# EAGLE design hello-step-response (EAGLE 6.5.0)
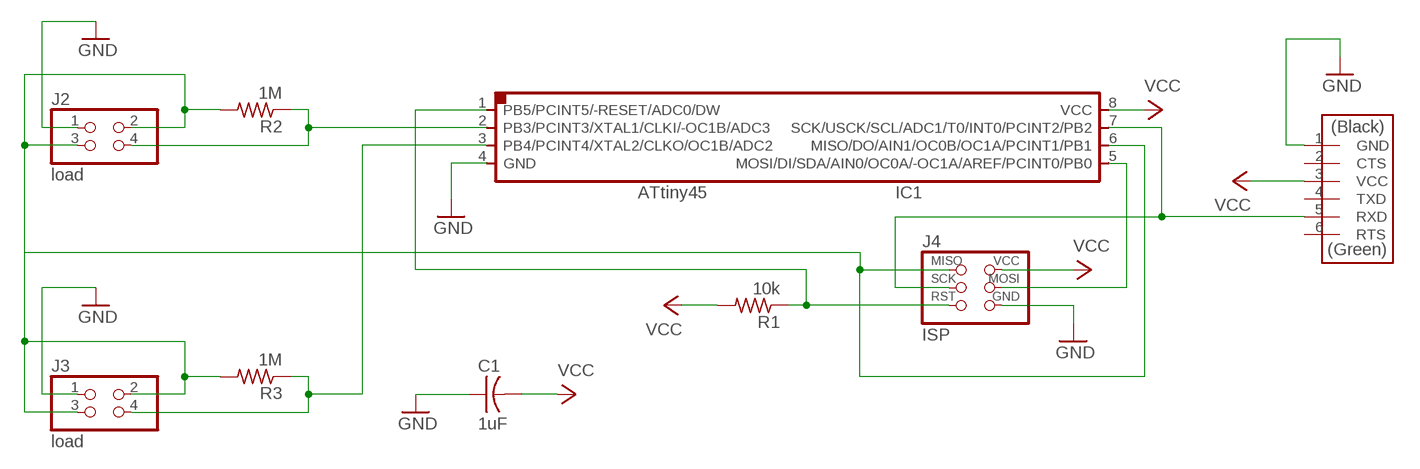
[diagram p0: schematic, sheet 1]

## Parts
C1  1uF  CAP-US1206FAB  [C1206FAB]
IC1  ATTINY45  ATTINY45SI  [SOIC8]
J1  FTDI  FTDI-SMD-HEADER  [1X06SMD]
J2  load  PINHD-2X2-SMD  [2X02SMD]
J3  load  PINHD-2X2-SMD  [2X02SMD]
J4  ISP  AVRISPSMD  [2X03SMD]
R1  10k  RES-US1206FAB  [R1206FAB]
R2  1M  RES-US1206FAB  [R1206FAB]
R3  1M  RES-US1206FAB  [R1206FAB]

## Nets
GND: C1.1 IC1.4(GND) J1.1(GND) J2.1 J3.1 J4.6(GND)
MISO: IC1.6(MISO/DO/AIN1/OC0B/OC1A/PCINT1/PB1) J2.2 J2.3 J3.2 J3.3 J4.1(MISO) R2.2 R3.2
MOSI: IC1.5(MOSI/DI/SDA/AIN0/OC0A/-OC1A/AREF/PCINT0/PB0) J4.4(MOSI)
N$5: IC1.2(PB3/PCINT3/XTAL1/CLKI/-OC1B/ADC3) J2.4 R2.1
N$6: IC1.3(PB4/PCINT4/XTAL2/CLKO/OC1B/ADC2) J3.4 R3.1
RST: IC1.1(PB5/PCINT5/-RESET/ADC0/DW) J4.5(RST) R1.1
SCK: IC1.7(SCK/USCK/SCL/ADC1/T0/INT0/PCINT2/PB2) J1.5(RXD) J4.3(SCK)
VCC: C1.2 IC1.8(VCC) J1.3(VCC) J4.2(VCC) R1.2
Unconnected: J1.2(CTS) J1.4(TXD) J1.6(RTS)

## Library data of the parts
C1 = fab:CAP-US
IC1 = fab:ATTINY45
J1 = fab:FTDI-SMD-HEADER
J2 J3 = fab:PINHD-2X2-SMD
J4 = fab:AVRISP
R1-R3 = fab:RES-US: Resistor (US Symbol)

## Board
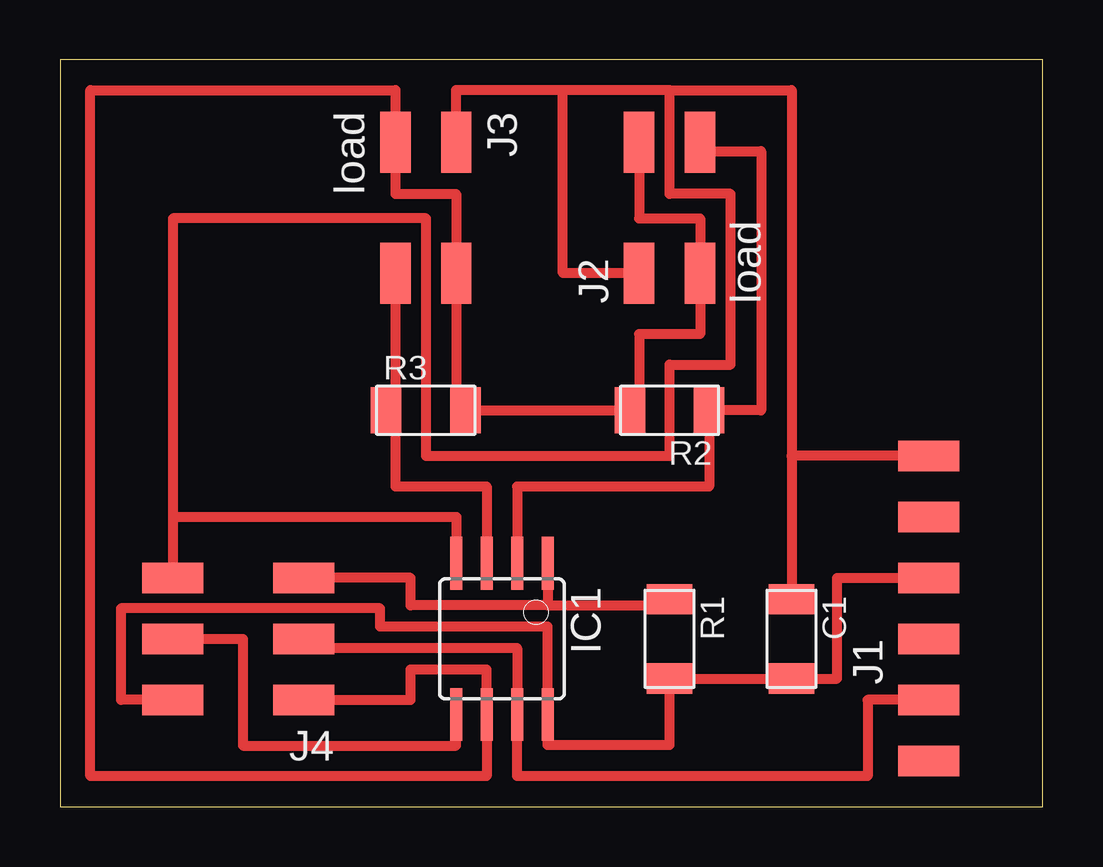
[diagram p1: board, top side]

Size 40.95 x 31.1 mm. Coordinates in mm from the lower left corner, seen from the top.
Outline: 0,0 40.95,0 40.95,31.1 0,31.1 0,0
Copper layers (1*16): Top 0.035mm / dielectric 1.5mm / Bottom 0.035mm
Design rules "design-rules-fablab": minimum track width 18mil, minimum drill 24mil, track to track 0.4mm, track to pad 0.4mm, pad to pad 0.4mm, via to via 0.4mm, smd to smd 8mil, copper to edge 1mil, drill to drill 8mil, minimum pad ring 10mil, minimum via ring 8mil, stop-mask expansion 4mil, vias tented up to drill 0mil, thermal gap 10mil

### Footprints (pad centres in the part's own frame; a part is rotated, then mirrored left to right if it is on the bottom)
C1206FAB = smd 1.27 x 1.905: 1 -1.651,0; 2 1.651,0
SOIC8 = smd 0.5 x 2.2: 1 -1.905,-3.154; 2 -0.645,-3.154; 3 0.625,-3.154; 4 1.895,-3.154; 5 1.905,3.154; 6 0.635,3.154; 7 -0.635,3.154; 8 -1.905,3.154
1X06SMD = smd 2.54 x 1.27: 1 0,6.35; 2 0,3.81; 3 0,1.27; 4 0,-1.27; 5 0,-3.81; 6 0,-6.35
2X02SMD = smd 2.54 x 1.27: 1 -2.54,1.27; 2 2.92,1.27; 3 -2.54,-1.27; 4 2.92,-1.27
2X03SMD = smd 2.54 x 1.27: 1 -2.54,2.54; 2 2.92,2.54; 3 -2.54,0; 4 2.92,0; 5 -2.54,-2.54; 6 2.92,-2.54
R1206FAB = smd 1.27 x 1.905: 1 -1.651,0; 2 1.651,0

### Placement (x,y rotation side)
C1  30.48,6.99 270 top
IC1  18.41,6.99 180 top
J1  36.2,8.26 0 top
J2  25.4,24.76 90 top
J3  15.24,25.15 270 top
J4  7.62,6.99 180 top
R1  25.4,6.99 270 top
R2  25.4,16.51 180 top
R3  15.24,16.51 0 top

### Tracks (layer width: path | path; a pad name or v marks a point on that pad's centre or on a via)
GND
  Top 0.406: 30.48,14.61 C1.1 | 4.7,12.06 16.52,12.06 IC1.4 | J3.1 16.51,29.84 20.95,29.84 | J1.1 30.48,14.61 | 25.4,29.84 20.95,29.84 | J2.1 20.95,22.22 20.95,29.84 | 25.4,29.84 25.4,25.53 27.94,25.53 27.94,18.41 25.4,18.41 25.4,14.61 15.24,14.61 15.24,24.51 4.7,24.51 4.7,12.06 | 25.4,29.84 30.48,29.84 30.48,14.61 | 4.7,12.06 J4.6
MISO
  Top 0.406: 9.53,4.45 J4.1 14.61,4.45 14.61,5.71 17.78,5.71 IC1.6 17.78,1.27 1.27,1.27 1.27,29.84 13.97,29.84 J3.3 13.97,25.53 16.51,25.53 J3.2 | 16.51,21.59 J3.2 | J3.2 16.51,16.51 R3.2 R2.2 24.13,16.51 24.13,19.68 26.67,19.68 J2.3 26.67,24.51 24.13,24.51 J2.2
MOSI
  Top 0.406: J4.4 7.62,6.99 7.62,2.54 16.51,2.54 IC1.5
N$5
  Top 0.406: J2.4 26.67,27.3 29.21,27.3 29.21,16.51 R2.1 27.05,13.34 19.05,13.34 IC1.2
N$6
  Top 0.406: J3.4 13.97,16.51 | R3.1 13.97,16.51 | 13.97,16.51 13.97,13.34 17.78,13.34 IC1.3
RST
  Top 0.406: 24.76,8.64 R1.1 25.4,8.38 20.32,8.38 | 24.76,8.64 24.76,8.26 | 24.76,8.89 24.76,8.64 | IC1.1 20.32,8.38 | 20.32,8.38 14.61,8.38 14.61,9.53 J4.5
SCK
  Top 0.406: J1.5 33.66,4.45 33.66,1.27 19.05,1.27 IC1.7 19.05,6.6 10.16,6.6 J4.3
VCC
  Top 0.406: J4.2 2.54,4.45 2.54,8.26 13.34,8.26 13.34,7.49 20.32,7.49 IC1.8 20.32,2.56 25.4,2.56 R1.2 C1.2 32.39,5.33 32.39,9.53 J1.3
